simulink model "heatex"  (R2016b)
settings: Solver=VariableStepAuto  StartTime=0.0  StopTime=10.0  RelTol=1e-3

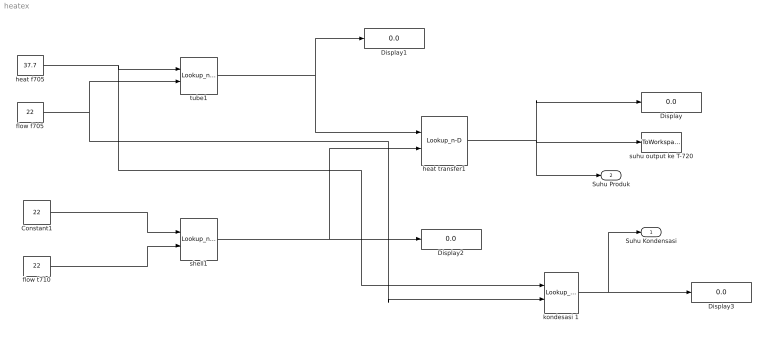
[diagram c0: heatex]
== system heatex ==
  Constant1 : Constant  Value=22
  Display{,1..3} (4 alike) : Display
  flow f705 : Constant  Value=22
  flow t710 : Constant  Value=22
  heat f705 : Constant  Value=37.7
  heat transfer1 : Lookup_n-D  BreakpointsForDimension1=[20,25,30]  BreakpointsForDimension2=[22,23,28,32,34,36,38,39,40,41,42,43,44,45,46,47,48,49,50,51,52,53,54,55,56,57,58,59,60,61,62]  Table=reshape([28,30,33,29,31,34,29,31,34,30,32,35,31,33,36,31,34,36,31,34,37,32,34,38,32,35,39,33,35,40,33,36,40,34,36,41,35,37,41,35,37,42,36,38,43,37,38,44,37,39,45,37,39,45,38,40,45,38,40,46,38,41,47,38,41,48,38,42,49,38,42,50,38,43,50,39,43,51,39,44,52,39,44,52,39,45,53,39,46,54,39,47,55],3,31)  InternalRulePriority=Speed  RndMeth=Simplest
  kondesasi 1 : Lookup_n-D  BreakpointsForDimension1=[37.7,38.1,38.2,38.4,38.5,38.6,38.7,38.9,40,40.1,40.2,40.3,40.4,40.5,40.6,40.7,40.8,40.9,41,41.1,41.2,41.3,41.4,41.5,41.6,41.7,41.8,41.9,42,42.1,42.2,42.3,42.4,42.5,42.6,42.7,42.8]  BreakpointsForDimension2=[21,22,27,28,32,34,35,37,38,39,40,41,42,43,45,46,48,49,50,51,52,53,54,55,56,57,58,59,60,61,62,63,64,65,66,67,68]  Table=reshape([28,0,0,0,0,0,0,0,0,0,0,0,0,0,0,0,0,0,0,0,0,0,0,0,0,0,0,0,0,0,0,0,0,0,0,0,0,0,28,0,0,0,0,0,0,0,0,0,0,0,0,0,0,0,0,0,0,0,0,0,0,0,0,0,0,0,0,0,0,0,0,0,0,0,0,0,28,0,0,0,0,0,0,0,0,0,0,0,0,0,0,0,0,0,0,0,0,0,0,0,0,0,0,0,0,0,0,0,0,0,0,0,0,0,28,0,0,0,0,0,0,0,0,0,0,0,0,0,0,0,0,0,0,0,0,0,0,0,0,0,0,0,0,0,0,0,0,0,0,0,0,0,28,0,0,0,0,0,0,0,0,0,0,0,0,0,0,0,0,0,0,0,0,0,0,0,0,0,0,0,0,0,0,0,0,0,0,0,0,0,28,0,0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  InternalRulePriority=Speed  RndMeth=Simplest
  shell1 : Lookup_n-D  BreakpointsForDimension1=[22,23,24,25,26,27,28,29,30,31,32,33,34,35,36,37,38,39,40,41,42,43,44,45,46,47,48,49,50,51]  BreakpointsForDimension2=[20,30,40]  Table=reshape([20,20,20,20,20,20,20,20,20,20,20,20,20,20,20,20,20,20,20,20,20,20,20,20,20,20,20,20,20,20,30,30,30,30,30,30,30,30,30,30,30,30,30,30,30,30,30,30,30,30,30,30,30,30,30,30,30,30,30,30,40,40,40,40,40,40,40,40,40,40,40,40,40,40,40,40,40,40,40,40,40,40,40,40,40,40,40,40,40,40],30,3)  InternalRulePriority=Speed  RndMeth=Simplest
  suhu output ke T-720 : ToWorkspace  VariableName=simout  SaveFormat=Timeseries  SampleTime=-1
  tube1 : Lookup_n-D  BreakpointsForDimension1=[37.7,38.2,38.6,39.1,39.6,40,40.2,40.4,40.9,41,41.1,41.2,41.3,41.4,41.5,41.6,41.7,41.8]  BreakpointsForDimension2=[50.5,60.5,65.5]  Table=reshape([20,20,24,24,25,26,26,27,28,29,29,30,31,32,32,33,34,34,21,23,23,23,25,26,28,29,29,30,31,33,35,35,35,36,36,37,22,28,28,32,34,36,38,39,39,40,41,43,44,45,46,47,48,48],18,3)  InternalRulePriority=Speed  RndMeth=Simplest
  Suhu Kondensasi : Outport
  Suhu Produk : Outport  Port=2
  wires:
  Constant1/1 -> shell1/1
  tube1/1 -> Display1/1, heat transfer1/1
  shell1/1 -> heat transfer1/2, Display2/1
  flow t710/1 -> shell1/2
  heat transfer1/1 -> Suhu Produk/1, suhu output ke T-720/1, Display/1
  kondesasi 1/1 -> Suhu Kondensasi/1, Display3/1
  heat f705/1 -> kondesasi 1/1, tube1/1
  flow f705/1 -> kondesasi 1/2, tube1/2
